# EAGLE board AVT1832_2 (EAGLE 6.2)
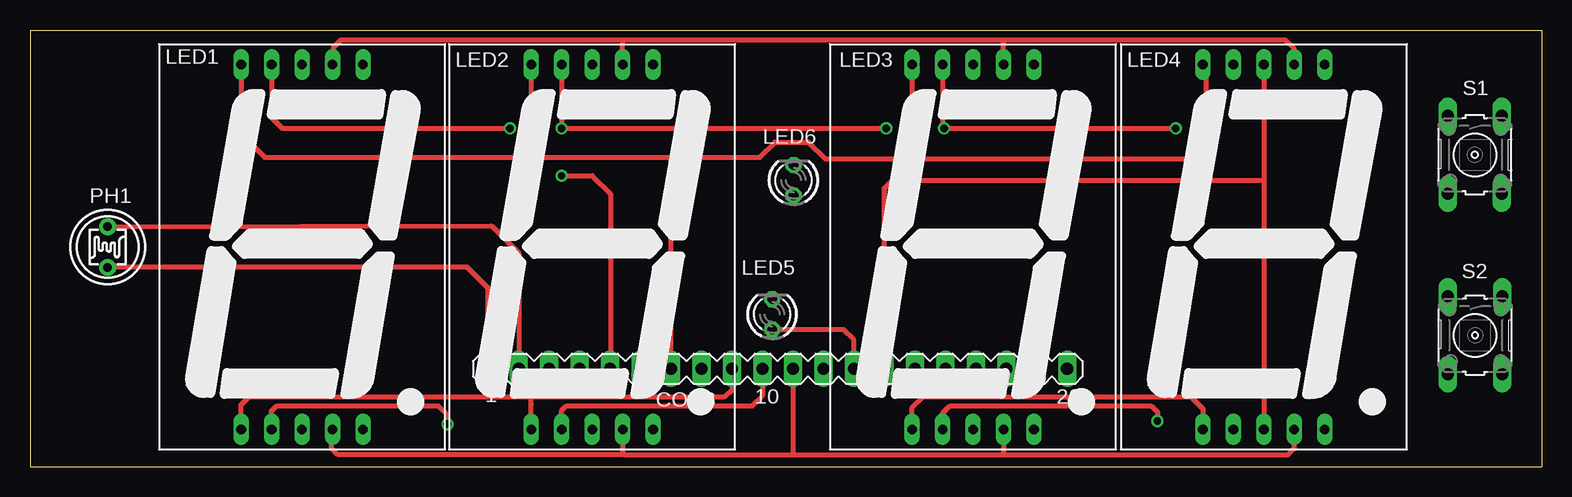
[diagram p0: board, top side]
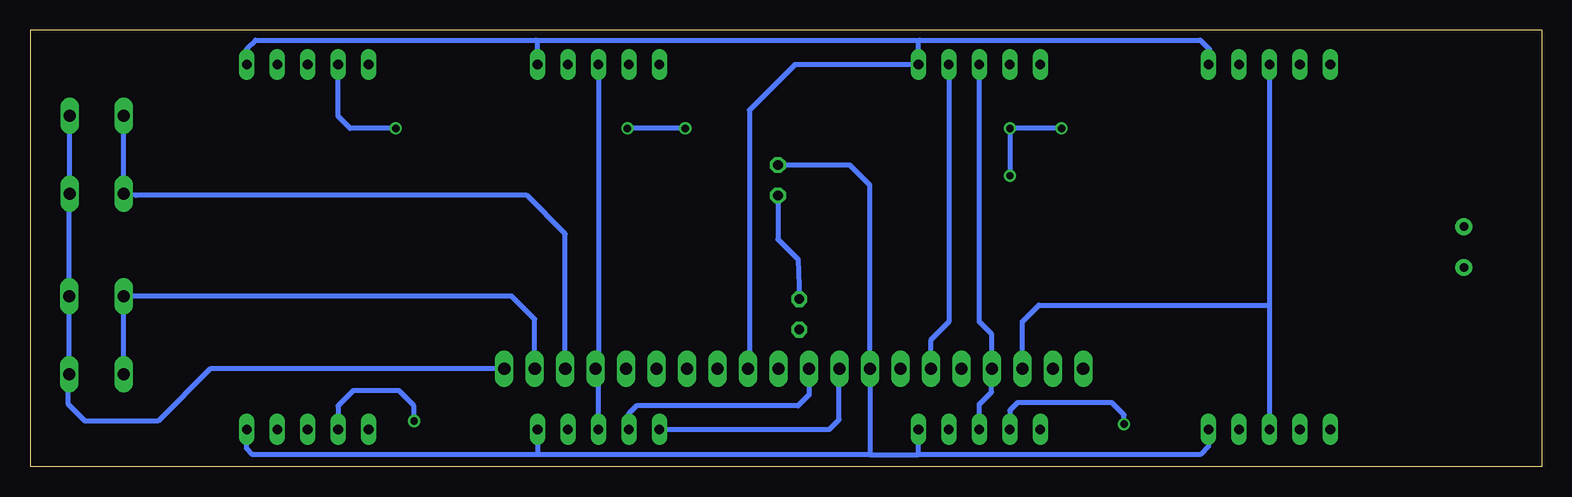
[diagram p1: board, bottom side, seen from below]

Size 126 x 36.4 mm. Coordinates in mm from the lower left corner, seen from the top.
Outline: 0,0 126,0 126,36.4 0,36.4 0,0
Copper layers (1*16): Top 0.035mm / dielectric 1.5mm / Bottom 0.035mm
Design rules: minimum track width 10mil, minimum drill 24mil, track to track 8mil, track to pad 8mil, pad to pad 8mil, via to via 8mil, smd to smd 8mil, copper to edge 40mil, drill to drill 8mil, minimum pad ring 10mil, minimum via ring 8mil, stop-mask expansion 4mil, vias tented up to drill 0mil, thermal gap 10mil

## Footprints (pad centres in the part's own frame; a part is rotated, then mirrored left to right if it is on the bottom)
MA20-1 = drill 1.016 long: 1 -24.13,0; 2 -21.59,0; 3 -19.05,0; 4 -16.51,0; 5 -13.97,0; 6 -11.43,0; 7 -8.89,0; 8 -6.35,0; 9 -3.81,0; 10 -1.27,0; 11 1.27,0; 12 3.81,0; 13 6.35,0; 14 8.89,0; 15 11.43,0; 16 13.97,0; 17 16.51,0; 18 19.05,0; 19 21.59,0; 20 24.13,0
SA10-21 = drill 0.8 long: 1 -5.08,-15.2; 2 -2.54,-15.2; 3 0,-15.2; 4 2.54,-15.2; 5 5.08,-15.2; 6 -5.08,15.2; 7 -2.54,15.2; 8 0,15.2; 9 2.54,15.2; 10 5.08,15.2
LED3MM = drill 0.813 octagon: A -1.27,0; K 1.27,0
T0-46-A10XX = drill 0.7 pad 1.4: 1 -1.7,0; 2 1.7,0
B3F-10XX = drill 1.016 long: 1 -3.251,2.261; 2 3.251,2.261; 3 -3.251,-2.261; 4 3.251,-2.261

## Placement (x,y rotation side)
CON3  [MA20-1]  62.33,8.16 0 top
LED1  7-SEG_SA10-21  [SA10-21]  22.68,18.32 0 top
LED2  7-SEG_SA10-21  [SA10-21]  46.86,18.32 0 top
LED3  7-SEG_SA10-21  [SA10-21]  78.61,18.32 0 top
LED4  7-SEG_SA10-21  [SA10-21]  102.85,18.32 0 top
LED5  [LED3MM]  61.87,12.7 90 top
LED6  [LED3MM]  63.65,23.88 90 top
PH1  A1050_09  [T0-46-A10XX]  6.47,18.31 270 top
S1  [B3F-10XX]  120.44,25.99 270 top
S2  [B3F-10XX]  120.46,10.96 270 top

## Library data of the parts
CON3 = con-lstb; OC_FARNELL: unknown; OC_NEWARK: unknown
LED1-LED4 = display-kingbright2; OC_FARNELL: unknown; OC_NEWARK: unknown
LED5 LED6 = led
PH1 = photo-elements
S1 S2 = switch-omron; MPN: B3F-1000; OC_FARNELL: 176432; OC_NEWARK: 36M3542

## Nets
A: CON3.5 LED1.7 LED2.7 LED3.7 LED4.7
A1: CON3.3 LED1.3 LED1.8
A2: CON3.4 LED2.3 LED2.8
A3: CON3.17 LED3.3 LED3.8
A4: CON3.14 LED4.3 LED4.8
A5: CON3.13 LED5.A
B: CON3.7 LED1.6 LED2.6 LED3.6 LED4.6
C: CON3.11 LED1.4 LED2.4 LED3.4 LED4.4
D: CON3.10 LED1.2 LED2.2 LED3.2 LED4.2
DP: CON3.8 LED1.5 LED2.5 LED3.5 LED4.5 LED6.K
E: CON3.9 LED1.1 LED2.1 LED3.1 LED4.1
F: CON3.6 LED1.9 LED2.9 LED3.9 LED4.9
G: CON3.12 LED1.10 LED2.10 LED3.10 LED4.10
GND: CON3.20 S1.1 S1.2 S2.1 S2.2
N$1: LED5.K LED6.A
N$2: CON3.1 PH1.2
N$3: CON3.2 PH1.1
S1: CON3.18 S1.3 S1.4
S2: CON3.19 S2.3 S2.4

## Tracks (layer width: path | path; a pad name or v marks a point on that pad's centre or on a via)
A  (via drill 0.6)
  Top 0.406: v40.01,28.19 21.03,28.19 20.14,29.08 LED1.7 | v71.37,28.19 v44.32,28.19 v44.32,28.2 LED2.7 | v95.5,28.19 v76.2,28.19 76.07,28.32 LED3.7 | v44.32,24.26 46.86,24.26 48.39,22.73 48.39,8.19 CON3.5 | LED1.7
  Bottom 0.406: v40.01,28.19 v44.32,28.19 v44.32,24.26 | v71.37,28.19 v76.2,28.19 | v95.5,28.19 99.31,28.19 100.33,29.21 100.33,33.5 LED4.7
A1
  Bottom 0.406: LED1.8 22.68,13.46 | 22.68,13.46 LED1.3 | CON3.3 43.28,12.09 41.91,13.46 22.68,13.46
A2
  Bottom 0.406: LED2.3 46.86,5.21 45.85,6.22 45.85,8.13 CON3.4 45.82,11.02 46.86,12.06 LED2.8
A3
  Bottom 0.406: LED3.8 78.61,8.39 CON3.17 78.61,7.93 LED3.3
A4
  Top 0.406: CON3.14 71.22,23.22 71.88,23.88 102.87,23.88 | 102.87,23.88 102.87,3.14 LED4.3 | LED4.8 102.85,23.89 102.87,23.88
  Bottom 0.406: LED4.3 102.85,2.52 102.74,2.41 102.74,3.01 LED4.3
A5
  Top 0.406: CON3.13 68.68,10.57 67.82,11.43 LED5.A
B
  Top 0.406: LED1.6 17.6,27.74 19.56,25.78 41.91,25.78 | 41.91,25.78 53.47,25.78 | 53.47,25.78 60.83,25.78 62.1,27.05 64.9,27.05 66.29,25.65 73.53,25.65 | 73.53,25.65 96.39,25.65 98.04,27.3 98.04,33.25 LED4.6 | LED3.6 73.53,25.66 73.53,25.65 | LED2.6 41.78,25.91 41.91,25.78 | CON3.7 53.44,25.76 53.47,25.78
C
  Top 0.406: 49.53,1.02 25.65,1.02 25.15,1.52 25.15,3.04 LED1.4 | LED2.4 49.4,1.15 49.53,1.02 | 49.53,1.02 63.5,1.02 | 63.5,1.02 81.03,1.02 | 81.03,1.02 104.9,1.02 105.41,1.52 105.41,3.1 LED4.4 | LED3.4 81.15,1.14 81.03,1.02 | CON3.11 63.6,1.12 63.5,1.02
D  (via drill 0.6)
  Top 0.406: LED2.2 44.32,4.7 44.7,5.08 60.2,5.08 61.09,5.97 61.09,8.13 CON3.10 | LED1.2 20.14,4.65 20.57,5.08 34.04,5.08 34.8,4.32 v34.8,3.56 | LED3.2 76.07,4.44 76.71,5.08 93.47,5.08 93.98,4.57 v93.98,3.81
  Bottom 0.406: v34.8,3.56 34.8,4.32 35.81,5.33 43.68,5.33 44.32,4.7 LED2.2 | CON3.10 61.06,5.99 61.98,5.08 75.44,5.08 76.07,4.45 LED3.2 | v93.98,3.81 93.98,5.08 95.25,6.35 99.06,6.35 100.33,5.08 100.33,3.14 LED4.2
DP
  Bottom 0.406: LED6.K 57.66,25.15 55.98,23.47 CON3.8 55.98,1.04 56.01,1.02 | LED1.5 27.76,1.7 28.45,1.02 51.94,1.02 | 51.94,1.02 LED2.5 | 56.01,1.02 51.94,1.02 | 56.01,1.02 83.82,1.02 | 83.82,1.02 107.44,1.02 107.95,1.52 107.95,3.1 LED4.5 | LED3.5 83.69,1.15 83.82,1.02
E
  Top 0.406: LED2.1 41.78,5.2 41.78,5.84 | 41.78,5.84 57.91,5.84 58.55,6.48 58.55,8.13 CON3.9 | LED1.1 17.6,5.16 18.29,5.84 41.78,5.84 | LED3.1 73.53,4.95 74.42,5.84 96.77,5.84 97.79,4.83 97.79,3.14 LED4.1
  Bottom 0.406: LED3.1 59.36,3.12 58.55,3.94 58.55,8.13 CON3.9
F
  Top 0.406: LED4.9 105.39,34.82 104.65,35.56 81.28,35.56 | 81.28,35.56 49.28,35.56 | 49.28,35.56 25.91,35.56 25.27,34.92 25.27,33.57 LED1.9 | LED2.9 49.4,35.44 49.28,35.56 | LED3.9 81.15,35.43 81.28,35.56
  Bottom 0.406: LED2.9 49.4,12.07 50.93,10.54 50.93,8.19 CON3.6
G
  Bottom 0.406: LED4.10 107.93,34.82 107.19,35.56 83.82,35.56 | 83.82,35.56 51.82,35.56 | 51.82,35.56 28.45,35.56 27.69,34.8 27.69,33.6 LED1.10 | 51.82,35.56 51.94,35.44 LED2.10 62.24,33.52 66.04,29.72 66.04,8.26 CON3.12 | LED3.10 83.69,35.43 83.82,35.56
GND
  Bottom 0.406: S1.1 S1.2 122.72,22.72 S2.1 S2.2 122.81,7.62 122.81,5.21 121.41,3.81 115.32,3.81 110.97,8.16 CON3.20
N$1
  Bottom 0.406: LED6.A 63.65,18.95 61.98,17.27 LED5.K
N$2
  Top 0.406: CON3.1 38.2,14.88 36.45,16.64 6.35,16.64 PH1.2
N$3
  Top 0.406: PH1.1 38.48,20.07 40.77,17.78 40.77,8.26 CON3.2
S1
  Bottom 0.406: CON3.18 81.38,19.41 84.58,22.61 117.17,22.61 S1.4 S1.3
S2
  Bottom 0.406: CON3.19 83.92,12.29 85.85,14.22 118.18,14.22 S2.3 118.24,14.21 118.24,7.62 118.2,7.66 S2.4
